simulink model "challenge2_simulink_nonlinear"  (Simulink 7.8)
settings: Solver=ode45  StartTime=0.0  StopTime=5.0  RelTol=1e-3
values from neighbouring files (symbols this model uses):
  g = 9.8    [challenge2_CST_solution.m]
  l = 2.5    [challenge2_CST_solution.m]
  m = 0.75    [challenge2_CST_solution.m]

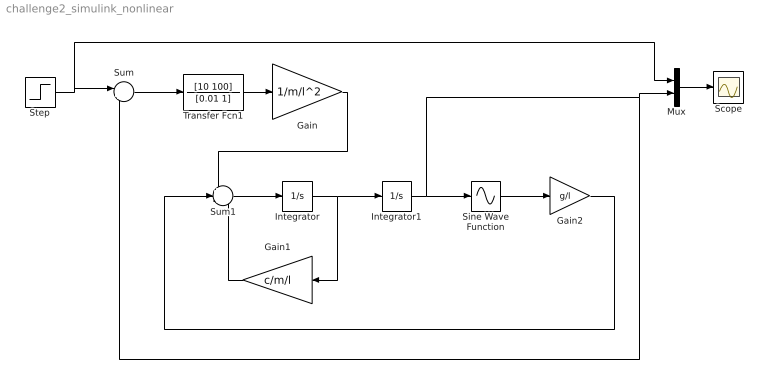
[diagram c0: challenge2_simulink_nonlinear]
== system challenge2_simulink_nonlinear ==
  Gain : Gain  Gain=1/m/l^2
  Gain1 : Gain  Gain=c/m/l
  Gain2 : Gain  Gain=g/l
  Integrator : Integrator
  Integrator1 : Integrator
  Mux : Mux  Inputs=2
  Scope : Scope
  Sine Wave Function : Sin  TimeSource=Use external signal  Samples=100  SampleTime=0
  Step : Step  After=45*pi/90  SampleTime=0
  Sum : Sum  Inputs=|+-
  Sum1 : Sum  Inputs=+--
  Transfer Fcn1 : TransferFcn  Numerator=[10 100]  Denominator=[0.01 1]
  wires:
  Mux/1 -> Scope/1
  Transfer Fcn1/1 -> Gain/1
  Sum/1 -> Transfer Fcn1/1
  Step/1 -> Mux/1, Sum/1
  Integrator/1 -> Integrator1/1, Gain1/1
  Gain/1 -> Sum1/1
  Sum1/1 -> Integrator/1
  Gain1/1 -> Sum1/3
  Integrator1/1 -> Mux/2, Sum/2, Sine Wave Function/1
  Gain2/1 -> Sum1/2
  Sine Wave Function/1 -> Gain2/1
